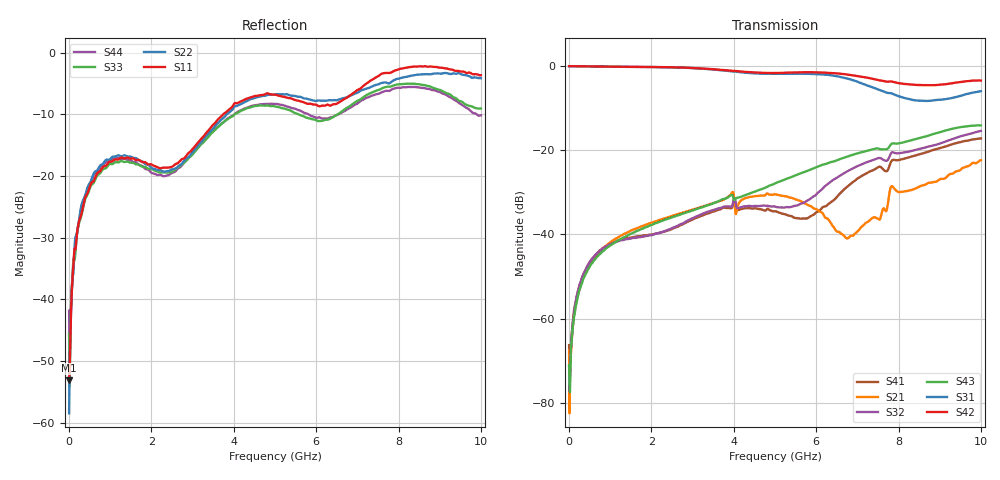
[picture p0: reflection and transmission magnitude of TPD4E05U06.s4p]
! Created Wed Sep 27 11:26:31 2017
# hz S ma R 50
! 4 Port Network Data from SP1.SP block
! freq  magS11  angS11  magS12  angS12  magS13  angS13  magS14  angS14
!  magS21  angS21  magS22  angS22  magS23  angS23  magS24  angS24
!  magS31  angS31  magS32  angS32  magS33  angS33  magS34  angS34
!  magS41  angS41  magS42  angS42  magS43  angS43  magS44  angS44
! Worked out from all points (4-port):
!   1001 points, 300 kHz to 10 GHz, reference 50 ohm
!   strongest paths, dB at 300 kHz, 2.5 GHz, 5 GHz, 7.5 GHz, 10 GHz:
!     S42: 0.0, -0.3, -1.6, -3.3, -3.4
!     S31: 0.0, -0.3, -1.8, -5.5, -5.9
!     S43: -71.1, -35.9, -27.9, -19.6, -14.1
!     S32: -71.4, -38.5, -33.4, -21.9, -15.4
!     S21: -67.6, -35.6, -30.4, -36.3, -22.4
!     S41: -66.3, -38.7, -34.5, -24.0, -17.2
!   lowest |S11| = -53.1 dB at 300 kHz (marker M1), VSWR 1.00, Z = 49.9 - j0.215 ohm
!   |S11| at or under -10 dB: start of sweep to 3.74 GHz
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300000  0.002212 -103.7  0.0001077 -102.0  1.001 0.3  0.0002531 -18.9
        0.0004168 68.6  0.001189 107.4  9.044e-05 171.4  0.9992 -0.2
        0.9998 -0.3  0.0002694 21.9  0.005265 108.2  0.0001747 -64.8
        0.0004838 86.7  1 -0.6  0.0002792 93.8  0.008096 98.6
1.903e8  0.03427 -71.6  0.001719 108.9  0.9996 -1.1  0.0019 85.6
         0.001715 106.4  0.03418 -68.1  0.001905 85.8  0.9991 -1.2
         0.9988 -1.2  0.001865 86.7  0.03401 -115.4  0.001635 65.4
         0.001871 87.3  0.9982 -1.2  0.001646 65.8  0.03442 -110.4
8.903e8  0.121 8.6  0.00734 171.2  0.9889 -4.6  0.007243 75.5
         0.007333 171.1  0.135 7.0  0.007169 80.3  0.9866 -4.6
         0.988 -4.6  0.007192 80.0  0.1157 158.8  0.006716 -16.7
         0.007232 75.6  0.9858 -4.6  0.006786 -16.5  0.13 161.5
6.6103e9  0.4061 -70.3  0.01007 -2.4  0.7412 -31.1  0.03188 142.4
          0.01019 -1.8  0.4252 -45.0  0.05124 148.8  0.811 -25.4
          0.7404 -31.0  0.05123 149.0  0.3318 117.0  0.07976 53.0
          0.03184 142.3  0.8104 -25.4  0.07975 53.0  0.3267 137.4
8.2403e9  0.7646 97.4  0.03346 12.7  0.4078 -30.3  0.08249 107.6
          0.03309 12.5  0.6444 115.6  0.09629 111.5  0.6086 -36.7
          0.4074 -30.0  0.09633 111.8  0.5636 -80.7  0.1289 -155.5
          0.08249 107.7  0.6086 -36.5  0.1289 -155.6  0.5293 -54.4
9.1103e9  0.7509 179.4  0.04596 84.3  0.4032 -19.9  0.1102 95.2
          0.04607 83.6  0.6857 -161.5  0.1255 102.4  0.6092 -36.2
          0.4037 -19.8  0.1256 102.5  0.4796 -179.4  0.1711 105.5
          0.11 95.0  0.6072 -36.2  0.1705 105.2  0.4624 -139.6
1e10  0.6584 -87.9  0.07672 -161.9  0.5039 -10.3  0.1379 82.3
      0.07629 -162.7  0.6229 -40.6  0.1701 104.6  0.6735 -30.0
      0.5046 -10.2  0.1701 104.8  0.3538 36.2  0.1978 -18.3
      0.1385 82.4  0.674 -29.9  0.1977 -18.4  0.311 93.7
